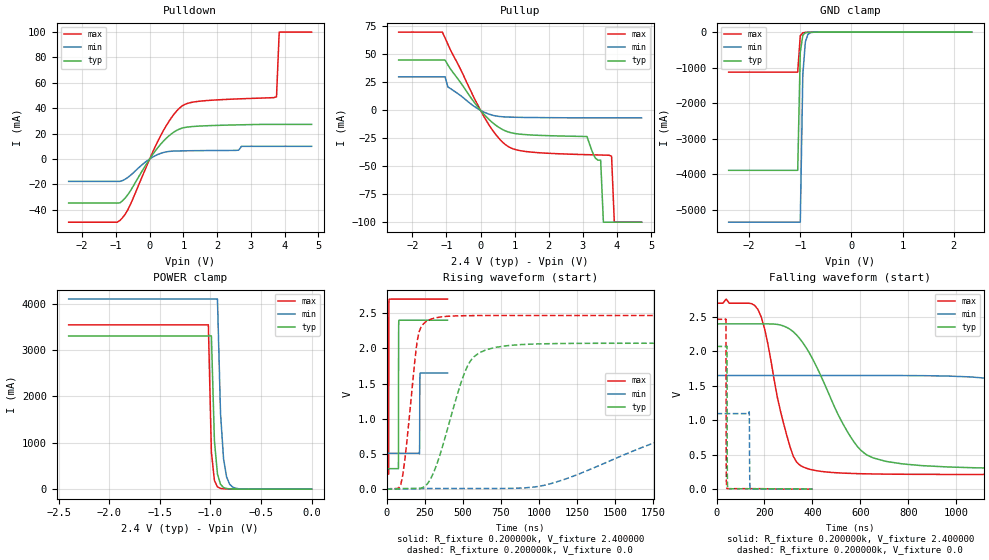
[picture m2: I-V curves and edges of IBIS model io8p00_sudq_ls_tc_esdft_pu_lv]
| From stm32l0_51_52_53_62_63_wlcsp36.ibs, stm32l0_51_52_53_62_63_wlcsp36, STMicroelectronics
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|   Model io8p00_sudq_ls_tc_esdft_pu_lv
[Model]  io8p00_sudq_ls_tc_esdft_pu_lv
Model_type I/O
Polarity   Non-Inverting
Enable   Active-Low
Vinl =   0.720000V
Vinh =   1.680000V
Vmeas =  1.200000V
Cref =   50.000000pF
Rref =   100.000000M
Vref =   0.0V
C_comp   2.242700pF   2.201100pF   2.288600pF
[Temperature Range]   25.000000   0.105000k   -40.000000
[Pullup Reference]   2.400000V   1.650000V   2.700000V
[Pulldown Reference]   0.0V   0.0V   0.0V
[POWER Clamp Reference]   2.400000V   1.650000V   2.700000V
[GND Clamp Reference]   0.0V   0.0V   0.0V
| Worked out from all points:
|   slope of the pulldown table from 0 to 0.36 V, typ, clamps not added: 28.4 ohm
|   slope of the pullup table from 0 to 0.36 V, typ, clamps not added: 32.2 ohm
|   GND clamp passes 1 mA (typ) near -0.65 V on its own axis
|   POWER clamp passes 1 mA (typ) near -0.63 V on its own axis
|   rising waveform, R_fixture 0.200000k, V_fixture 2.400000: 20-80 % time 631ps typ, 855ps min, 658ps max; typ from 0.292 V to 2.4 V
|   rising waveform, R_fixture 0.200000k, V_fixture 0.0: 20-80 % time 174ns typ, 838ns min, 69.6ns max; typ from 0.001 V to 2.07 V
|   falling waveform, R_fixture 0.200000k, V_fixture 2.400000: 20-80 % time 181ns typ, 739ns min, 90.4ns max; typ from 2.4 V to 0.292 V
|   falling waveform, R_fixture 0.200000k, V_fixture 0.0: 20-80 % time 752ps typ, 1.17ns min, 667ps max; typ from 2.07 V to 0.001 V
[Pulldown]
|Voltage   I(typ)   I(min)   I(max)
-2.4V     -34.71mA   -17.61mA   -49.77mA
-880mV    -34.55mA   -17.61mA   -48.41mA
-560mV    -24.66mA   -12.69mA   -35.31mA
240mV     8.893mA    3.542mA    13.9mA
560mV     17.98mA    5.931mA    29.16mA
880mV     23.58mA    6.388mA    40.03mA
1.44V     25.89mA    6.593mA    45.41mA
2.64V     26.92mA    7mA        47.38mA
2.72V     26.96mA    10mA       47.46mA
3.76V     27.3mA     10mA       49mA
3.84V     27.3mA     10mA       100mA
4.8V      27.3mA     10mA       100mA
[Pullup]
|Voltage   I(typ)   I(min)   I(max)
-2.4V     45mA       30mA       70mA
-1.12V    45mA       30mA       70mA
-960mV    40.7mA     21mA       59.3mA
80mV      -2.838mA   -1.261mA   -4.478mA
800mV     -19.2mA    -5.978mA   -32.18mA
3.12V     -23.45mA   -6.63mA    -39.62mA
3.36V     -42.53mA   -6.63mA    -39.81mA
3.52V     -44.5mA    -6.63mA    -39.93mA
3.6V      -100mA     -6.63mA    -40mA
3.84V     -100mA     -6.63mA    -41mA
3.92V     -100mA     -6.63mA    -100mA
4.72V     -100mA     -6.63mA    -100mA
[GND_clamp]
|Voltage   I(typ)   I(min)   I(max)
-2.4V     -3.892A    -5.353A    -1.127A
-1.05V    -3.892A    -5.353A    -1.127A
-1V       -568.8mA   -5.353A    -105.4mA
-950mV    -88.95mA   -1.19A     -18.03mA
-900mV    -18.15mA   -269.2mA   -8.959mA
-850mV    -6.699mA   -63.45mA   -6.568mA
-800mV    -4.014mA   -16.61mA   -4.858mA
-650mV    -1.043mA   -1.218mA   -1.146mA
2.35V     0A         0A         0A
[POWER_clamp]
|Voltage   I(typ)   I(min)   I(max)
-2.4V     3.303A     4.097A     3.542A
-1.02V    3.303A     4.097A     3.542A
-990mV    3.303A     4.097A     802.4mA
-960mV    1.032A     4.097A     186.5mA
-930mV    325.2mA    4.097A     47.6mA
-900mV    104.9mA    1.637A     15.79mA
-870mV    35.84mA    655.7mA    8.024mA
-840mV    13.94mA    263.9mA    5.676mA
-810mV    6.724mA    107.2mA    4.568mA
-780mV    4.1mA      44.41mA    3.772mA
-690mV    1.753mA    4.377mA    1.918mA
0V        0A         0A         0A
[Ramp]
| variable   typ   min   max
dV/dt_r  0.65094/0.30886u   0.19035/0.83514u   1.03799/0.14879u
dV/dt_f  0.75624/0.32503u   0.19656/0.85250u   1.13750/0.16128u
R_load = 50.000000
[Rising Waveform]
R_fixture= 0.200000k
V_fixture= 2.400000
V_fixture_min= 1.650000
V_fixture_max= 2.700000
|time   V(typ)   V(min)   V(max)
0s        291.9mV    510.4mV    213.7mV
14.01ns   291.9mV    510.4mV    221.4mV
15.22ns   291.9mV    510.4mV    2.513V
16.82ns   291.9mV    510.4mV    2.697V
77.68ns   290mV      510.4mV    2.7V
79.28ns   2.152V     510.4mV    2.7V
80.88ns   2.396V     510.4mV    2.7V
215.8ns   2.4V       502.1mV    2.7V
220.2ns   2.4V       1.647V     2.7V
400ns     2.4V       1.65V      2.7V
[Rising Waveform]
R_fixture= 0.200000k
V_fixture= 0.0
V_fixture_min= 0.0
V_fixture_max= 0.0
|time   V(typ)   V(min)   V(max)
0s        1.185mV    2.217mV    641.2uV
93.43ns   10.69mV    2.217mV    65.1mV
213.5ns   14.46mV    2.207mV    2.236V
293.6ns   167.6mV    10.06mV    2.417V
400.4ns   861.1mV    10.06mV    2.455V
560.6ns   1.85V      10.08mV    2.465V
880.9ns   2.054V     16.13mV    2.467V
2.015us   2.073V     834.6mV    2.467V
2.936us   2.073V     1.066V     2.467V
13.33us   2.073V     1.097V     2.467V
[Falling Waveform]
R_fixture= 0.200000k
V_fixture= 2.400000
V_fixture_min= 1.650000
V_fixture_max= 2.700000
|time   V(typ)   V(min)   V(max)
0s        2.4V       1.65V      2.7V
173.5ns   2.4V       1.65V      2.605V
320.3ns   2.285V     1.65V      477.7mV
520.5ns   993.4mV    1.65V      234.8mV
627.3ns   496.6mV    1.65V      223.1mV
854.2ns   342.9mV    1.648V     215.7mV
1.348us   298.5mV    1.506V     213.7mV
2.229us   292.1mV    720.4mV    213.7mV
2.99us    291.9mV    555mV      213.7mV
13.33us   291.9mV    510.4mV    213.7mV
[Falling Waveform]
R_fixture= 0.200000k
V_fixture= 0.0
V_fixture_min= 0.0
V_fixture_max= 0.0
|time   V(typ)   V(min)   V(max)
0s        2.073V     1.097V     2.467V
39.24ns   2.073V     1.097V     2.47V
40.44ns   2.073V     1.097V     429.3mV
42.84ns   2.072V     1.097V     11.91mV
43.64ns   2.071V     1.097V     9.248mV
45.25ns   163.4mV    1.097V     8.616mV
47.25ns   9.837mV    1.097V     8.572mV
136.5ns   6.456mV    1.122V     8.545mV
140.9ns   6.456mV    4.519mV    8.546mV
400ns     1.185mV    2.217mV    641.2uV
